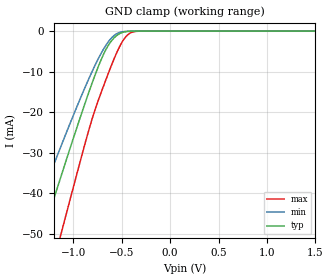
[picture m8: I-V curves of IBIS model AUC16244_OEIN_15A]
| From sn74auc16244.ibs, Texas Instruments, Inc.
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[Model]   AUC16244_OEIN_15A
Model_type  Input
Vinl=0.49
Vinh=1.04
| variable   typ   min   max
C_comp   2.54pF   2.10pF   2.92pF
[Temperature Range]   40   100   -40
| Ambient temperature   25   85   -40
[Voltage range]   1.5   1.4   1.6
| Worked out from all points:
|   GND clamp passes 1 mA (typ) near -0.55 V on its own axis
[GND Clamp]
| AUC16244_OEIN_15A
|   Voltage   I(typ)   I(min)   I(max)
-3.6V     -226.6mA   -190.3mA   -271.8mA
-1.465V   -61.48mA   -49.43mA   -80.77mA
-1.29V    -48.15mA   -38.43mA   -64.9mA
-1.13V    -36.11mA   -28.6mA    -50.37mA
-1.08V    -32.4mA    -25.59mA   -45.83mA
-815mV    -13.48mA   -10.49mA   -22.45mA
-695mV    -6.152mA   -4.773mA   -14.06mA
-575mV    -1.605mA   -1.034mA   -6.664mA
-500mV    -407.2uA   -207.5uA   -2.896mA
-435mV    -83.64uA   -40.42uA   -873uA
-310mV    -2.072uA   -1.331uA   -17.49uA
1.5V      165.9pA    259.7pA    172.1pA
